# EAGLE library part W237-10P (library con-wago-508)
WAGO SREW CLAMP
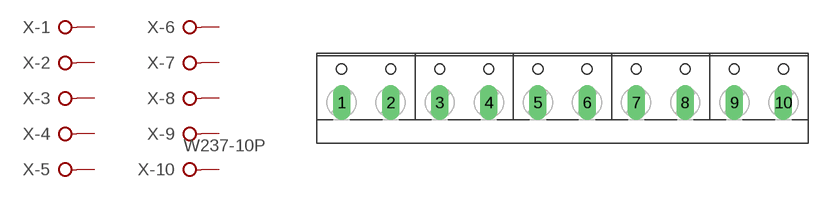
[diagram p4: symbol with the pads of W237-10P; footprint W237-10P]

Designator prefix X; gates -1=KL -2=KL -3=KL -4=KL -5=KL -6=KL -7=KL -8=KL -9=KL -10=KL+V

## W237-10P (OC_FARNELL: unknown; OC_NEWARK: unknown)  [W237-10P]
1  -1:KL  pas
2  -2:KL  pas
3  -3:KL  pas
4  -4:KL  pas
5  -5:KL  pas
6  -6:KL  pas
7  -7:KL  pas
8  -8:KL  pas
9  -9:KL  pas
10  -10:KL  pas

## Footprint W237-10P (pad centres in mm)
WAGO SREW CLAMP
drill 1.194 long: 1 -22.86,-0.635; 2 -17.78,-0.635; 3 -12.7,-0.635; 4 -7.62,-0.635; 5 -2.54,-0.635; 6 2.54,-0.635; 7 7.62,-0.635; 8 12.7,-0.635; 9 17.78,-0.635; 10 22.86,-0.635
